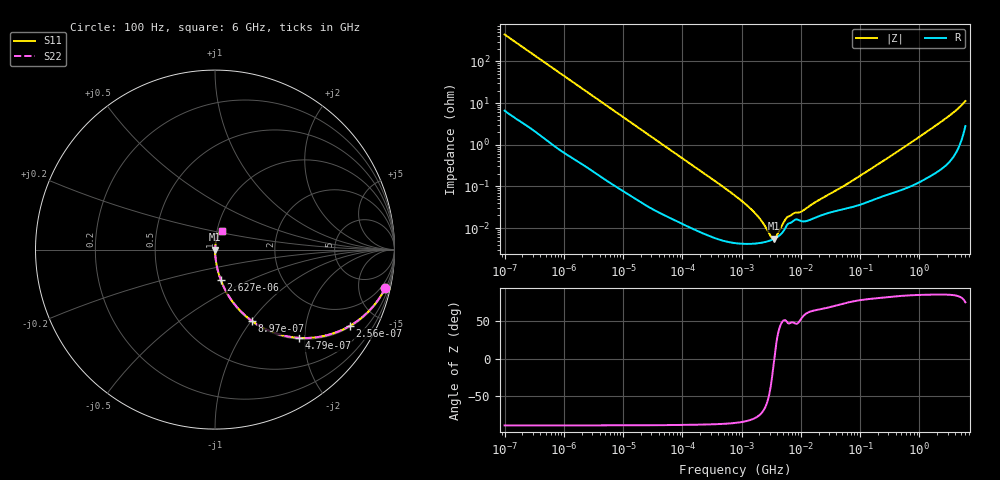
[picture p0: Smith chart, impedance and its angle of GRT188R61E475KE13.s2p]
!Murata Part Number: GRT188R61E475KE13
!These Parameters are Measured in Series Mode Connection
!Data Generated on Jun 19, 2026
!  o--ll--o
!Port1  Port2
!  o------o
!Operation Temp=25[degC], DC Bias Voltage=0[V]
!Freq. Start=100[Hz] Stop=6[GHz] 401[Steps]
# Hz S RI R 50
!Freq.(Hz) S11(Real) S11(Imag) S21(Real) S21(Imag) S12(Real) S12(Imag) S22(Real) S22(Imag)
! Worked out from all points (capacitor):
!   401 points, 100 Hz to 6 GHz, reference 50 ohm
!   read as one part in series: C = 3.58 uF near 109 Hz
!   lowest |Z| = 5.5 mohm at 3.55 MHz (marker M1)
!   series resonance near 3.562 MHz, so ESL is about 560 pH
!   S11 on the Smith chart (normalised r, x): 100 Hz: 1.13, -8.86; 256 Hz: 1.05, -3.49; 479 Hz: 1.03, -1.88; 897 Hz: 1.01, -1.01; 2.627 kHz: 1.01, -0.35; 6 GHz: 1.06, +0.22
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100  0.9486 -0.2134  0.0514 0.2134  0.0514 0.2134  0.9486 -0.2134
164  0.8772 -0.3209  0.1228 0.3209  0.1228 0.3209  0.8772 -0.3209
256  0.7495 -0.4258  0.2505 0.4258  0.2505 0.4258  0.7495 -0.4258
479  0.4686 -0.4917  0.5314 0.4917  0.5314 0.4917  0.4686 -0.4917
897  0.2058 -0.3973  0.7942 0.3973  0.7942 0.3973  0.2058 -0.3973
2008  0.0518 -0.2142  0.9482 0.2142  0.9482 0.2142  0.0518 -0.2142
2627  0.0317 -0.1678  0.9683 0.1678  0.9683 0.1678  0.0317 -0.1678
8047  0.0042 -0.057  0.9958 0.057  0.9958 0.057  0.0042 -0.057
40335  0.00037 -0.0116  0.9996 0.0116  0.9996 0.0116  0.00037 -0.0116
774597  4.37e-05 -0.000597  1 0.000597  1 0.000597  4.37e-05 -0.000597
1585629  4.2e-05 -0.000246  1 0.000246  1 0.000246  4.2e-05 -0.000246
2594782  4.67e-05 -8.86e-05  1 8.86e-05  1 8.86e-05  4.67e-05 -8.86e-05
3549919  5.5e-05 -9e-07  0.9999 9e-07  0.9999 9e-07  5.5e-05 -9e-07
4440638  6.77e-05 6.3e-05  0.9999 -6.3e-05  0.9999 -6.3e-05  6.77e-05 6.3e-05
6075234  0.000126 0.000138  0.9999 -0.000138  0.9999 -0.000138  0.000126 0.000138
7599586  0.000151 0.000168  0.9998 -0.000168  0.9998 -0.000168  0.000151 0.000168
1.039699e7  0.000145 0.000205  0.9999 -0.000205  0.9999 -0.000205  0.000145 0.000205
1.555665e7  0.000164 0.000336  0.9998 -0.000336  0.9998 -0.000336  0.000164 0.000336
5.960426e7  0.000295 0.00109  0.9997 -0.00109  0.9997 -0.00109  0.000295 0.00109
3.124326e8  0.000676 0.00503  0.9993 -0.00503  0.9993 -0.00503  0.000676 0.00503
2.450438e9  0.00407 0.037  0.9959 -0.037  0.9959 -0.037  0.00407 0.037
6e9  0.0379 0.1013  0.9621 -0.1013  0.9621 -0.1013  0.0379 0.1013
